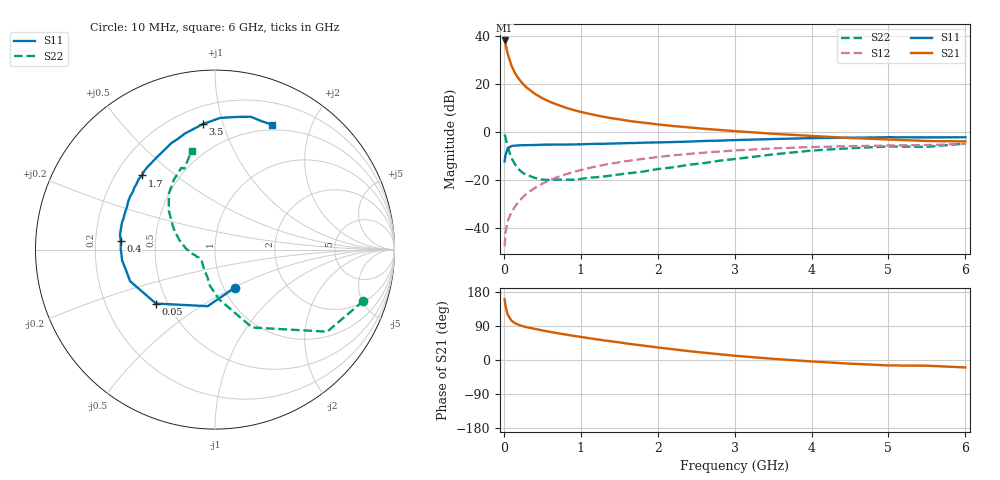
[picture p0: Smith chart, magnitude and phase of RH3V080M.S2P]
! SIEMENS Small Signal Semiconductors
! BFR106
! Si NPN RF Bipolar Junction Transistor in SOT23
! VCE = 3 V  IC = 80 mA
! Common Emitter S-Parameters:  August  1996
# GHz  S  MA  R  50
!  f  S11  S21  S12  S22
! GHz  MAG  ANG  MAG  ANG  MAG  ANG  MAG  ANG
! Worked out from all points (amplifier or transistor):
!   36 points, 10 MHz to 6 GHz, reference 50 ohm
!   highest |S21| = 38.1 dB at 10 MHz (marker M1)
!   |S21| within 3 dB of that: start of sweep to 32.21 MHz
!   unconditionally stable (mu >= 1): 180.8 MHz to 2.538 GHz; 5.353 GHz to end of sweep
!   at 250 MHz: K = 1.05, MAG = 22.2 dB, |S12| = -27.2 dB
!   at 1.4 GHz: K = 1.06, MAG = 7.9 dB, |S12| = -13.3 dB
!   at 6 GHz: K = 1.00, MAG = 0.4 dB, |S12| = -5.1 dB
!   S11 on the Smith chart (normalised r, x): 10 MHz: 1.13, -0.51; 50 MHz: 0.43, -0.32; 400 MHz: 0.31, +0.04; 1.7 GHz: 0.31, +0.38; 3.5 GHz: 0.31, +0.86; 6 GHz: 0.43, +1.47
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0.01  0.2397 -62.7  79.96 160.2  0.0041 78.1  0.8749 -19.1
0.02  0.3179 -97.4  69.32 144.7  0.0076 69.1  0.7744 -36.2
0.05  0.4457 -137.6  42.14 119.2  0.0137 61.3  0.4809 -64.5
0.1  0.5044 -159.5  23.7 103.7  0.0212 64.2  0.2778 -85.4
0.15  0.511 -168.4  16.17 96.5  0.0281 68.2  0.2033 -98.0
0.2  0.521 -173.5  12.3 92.2  0.0357 70.9  0.161 -104.9
0.25  0.5225 -177.6  9.854 88.8  0.0435 72.3  0.1367 -113.4
0.3  0.5253 179.8  8.243 86.4  0.0514 73.2  0.1256 -118.7
0.4  0.5272 174.6  6.235 82.2  0.0668 73.5  0.109 -128.7
0.5  0.536 171.0  5.005 78.1  0.0823 73.2  0.1001 -135.8
0.6  0.537 167.2  4.196 74.2  0.0979 72.1  0.0984 -140.3
0.7  0.5398 163.7  3.63 70.6  0.1137 71.2  0.0999 -145.0
0.9  0.5424 157.5  2.853 64.0  0.1438 68.2  0.0996 -153.7
1.1  0.553 151.1  2.377 57.8  0.1737 65.5  0.1095 -158.8
1.4  0.5666 142.5  1.912 49.2  0.2165 60.7  0.1222 -166.9
1.7  0.5806 134.6  1.618 40.8  0.2574 55.9  0.1404 -176.1
2.2  0.6083 122.2  1.312 28.3  0.3212 47.7  0.1808 171.2
2.8  0.6508 108.5  1.089 15.3  0.3856 37.9  0.2477 155.3
3.5  0.7027 95.5  0.906 3.1  0.4476 27.0  0.3358 140.0
4.5  0.7482 81.0  0.74 -9.7  0.4983 12.5  0.4519 120.5
5.5  0.7611 69.4  0.639 -15.1  0.5269 3.5  0.4832 110.7
6  0.7658 65.5  0.628 -19.6  0.5576 -3.4  0.5646 103.4
